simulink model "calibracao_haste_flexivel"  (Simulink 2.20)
settings: Solver=ode1  StartTime=0.0  StopTime=999999  FixedStep=0.01  RelTol=1e-3  AbsTol=1e-6
libraries: winlib x4

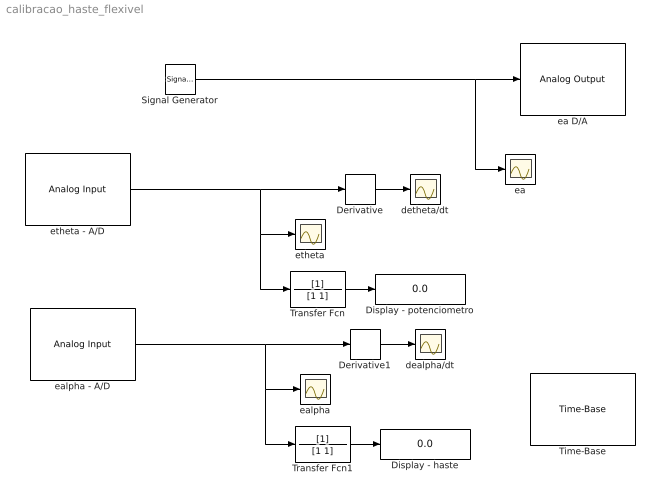
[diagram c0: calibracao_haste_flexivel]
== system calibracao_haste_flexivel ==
  Derivative : Derivative
  Derivative1 : Derivative
  Display - haste : Display
  Display - potenciometro : Display
  Signal Generator : SignalGenerator  WaveForm=square  Amplitude=0.5  Frequency=0.2  Units=Hertz
  Time-Base : winlib/Quanser Consulting MultiQ Series/Time-Base  baseAddr=0x320  irqLevel=9  clockSource=1
  Transfer Fcn : TransferFcn  Numerator=[1]  Denominator=[1 1]
  Transfer Fcn1 : TransferFcn  Numerator=[1]  Denominator=[1 1]
  dealpha/dt : Scope
  detheta/dt : Scope
  ea : Scope
  ea D/A : winlib/Quanser Consulting MultiQ Series/Analog Output  baseAddr=0x320  channels=[4]  initialOutputs=0  finalOutputs=0  sampleTime=str2num(get_param(bdroot, 'FixedStep'))
  ealpha : Scope
  ealpha - A/D : winlib/Quanser Consulting MultiQ Series/Analog Input  baseAddr=0x320  channels=[2]  sampleTime=str2num(get_param(bdroot, 'FixedStep'))
  etheta : Scope
  etheta - A/D : winlib/Quanser Consulting MultiQ Series/Analog Input  baseAddr=0x320  channels=[1]  sampleTime=str2num(get_param(bdroot, 'FixedStep'))
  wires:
  Derivative/1 -> detheta/dt/1
  Signal Generator/1 -> ea D/A/1, ea/1
  etheta - A/D/1 -> Derivative/1, etheta/1, Transfer Fcn/1
  Derivative1/1 -> dealpha/dt/1
  ealpha - A/D/1 -> Derivative1/1, ealpha/1, Transfer Fcn1/1
  Transfer Fcn1/1 -> Display - haste/1
  Transfer Fcn/1 -> Display - potenciometro/1
